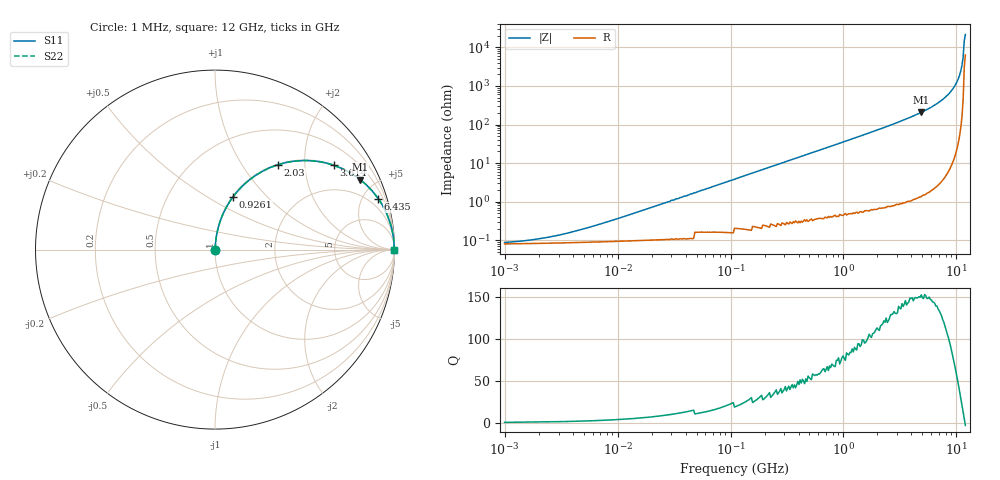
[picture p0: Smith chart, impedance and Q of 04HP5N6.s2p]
# MHz S MA R 50
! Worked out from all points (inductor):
!   408 points, 1 MHz to 12 GHz, reference 50 ohm
!   read as one part in series: L = 5.6 nH near 7.981 MHz
!   highest Q = 150 at 4.879 GHz (marker M1), where L = 6.73 nH
!   self-resonance near 11.73 GHz
!   S11 on the Smith chart (normalised r, x): 1 MHz: 1.00, +0.00; 926.1 MHz: 1.01, +0.65; 2.03 GHz: 1.01, +1.47; 3.614 GHz: 1.02, +2.80; 6.435 GHz: 1.04, +6.41; 12 GHz: open
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1  0.0007012 30.1  0.999 -0.0  0.999 -0.0  0.0007012 30.1
2.093  0.0009907 47.9  0.999 -0.0  0.999 -0.0  0.0009907 47.9
4.803  0.001851 65.7  0.999 -0.1  0.999 -0.1  0.001851 65.7
23.071  0.008181 81.9  0.999 -0.5  0.999 -0.5  0.008181 81.9
110.816  0.039 85.1  0.997 -2.2  0.997 -2.2  0.039 85.1
260.277  0.091 83.2  0.993 -5.2  0.993 -5.2  0.091 83.2
532.275  0.184 78.4  0.98 -10.6  0.98 -10.6  0.184 78.4
926.141  0.31 71.2  0.946 -18.1  0.946 -18.1  0.31 71.2
1403.083  0.446 62.9  0.89 -26.5  0.89 -26.5  0.446 62.9
2029.758  0.59 53.3  0.802 -36.2  0.802 -36.2  0.59 53.3
2556.642  0.683 46.4  0.725 -43.1  0.725 -43.1  0.683 46.4
3614.167  0.811 35.4  0.579 -54.2  0.579 -54.2  0.811 35.4
4878.67  0.898 25.8  0.435 -63.8  0.435 -63.8  0.898 25.8
6435.35  0.953 17.3  0.297 -72.3  0.297 -72.3  0.953 17.3
7391.073  0.972 13.2  0.229 -76.3  0.229 -76.3  0.972 13.2
8295.075  0.983 10.0  0.173 -79.5  0.173 -79.5  0.983 10.0
9097.259  0.99 7.4  0.128 -82.0  0.128 -82.0  0.99 7.4
9977.019  0.995 4.8  0.084 -84.2  0.084 -84.2  0.995 4.8
10448.31  0.997 3.5  0.062 -85.2  0.062 -85.2  0.997 3.5
10941.86  0.998 2.3  0.04 -85.7  0.04 -85.7  0.998 2.3
11726.24  0.999 0.4  0.006726 -77.9  0.006726 -77.9  0.999 0.4
12000  0.999 -0.3  0.004636 72.7  0.004636 72.7  0.999 -0.3
